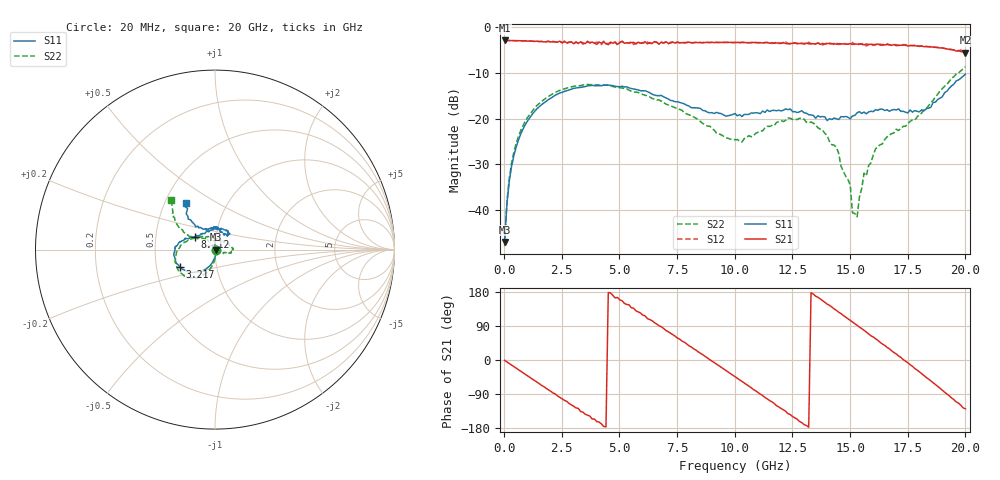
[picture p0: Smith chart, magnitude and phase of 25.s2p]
!Agilent Technologies,N5230A,US43500223,A.07.50.48
!Agilent N5230A: A.07.50.48
!Date: Sunday, September 13, 2015 17:37:15
!Correction: S11(Full 2 Port(1,2))
!S21(Full 2 Port(1,2))
!S12(Full 2 Port(1,2))
!S22(Full 2 Port(1,2))
!S2P File: Measurements: S11, S21, S12, S22:
# Hz S  dB  R 50
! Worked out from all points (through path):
!   201 points, 20 MHz to 20 GHz, reference 50 ohm
!   highest |S21| = -2.98 dB at 20 MHz (marker M1); lowest = -5.6 dB at 20 GHz (marker M2)
!   group delay of S21, straight-line fit = 116 ps
!   lowest |S11| = -46.9 dB at 20 MHz (marker M3), VSWR 1.01, Z = 50.4 - j0.124 ohm
!   |S11| at or under -10 dB: start of sweep to end of sweep
!   |S22| runs from -47.8 to -8.7 dB; largest |S21 - S12| = 0.042
!   S11 on the Smith chart (normalised r, x): 20 MHz: 1.01, -0.00; 3.217 GHz: 0.66, -0.14; 8.112 GHz: 0.79, +0.12; 20 GHz: 0.64, +0.37
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2e7  -46.90 -15.9  -2.98 -0.9  -2.97 -0.9  -47.81 -29.2
1.199e8  -38.58 -70.6  -2.98 -5.0  -2.98 -5.1  -38.16 -67.5
3.197e8  -30.45 -84.5  -3.01 -13.4  -3.00 -13.4  -29.74 -84.3
8.192e8  -22.27 -102.4  -3.07 -33.9  -3.07 -34.0  -21.53 -98.7
2.1179e9  -15.23 -133.2  -3.28 -86.9  -3.13 -86.2  -14.55 -123.2
3.2168e9  -13.25 -153.1  -3.57 -127.8  -3.68 -128.4  -12.86 -142.9
3.4166e9  -13.11 -156.6  -3.48 -137.4  -3.79 -137.6  -12.69 -145.8
5.1149e9  -12.95 177.9  -3.11 156.2  -3.21 156.1  -13.30 -175.9
6.7133e9  -15.00 159.4  -3.79 90.4  -3.71 90.0  -15.93 159.6
8.1119e9  -17.62 147.0  -3.46 34.3  -3.51 33.8  -19.35 139.9
9.011e9  -18.71 133.6  -3.37 -3.0  -3.39 -2.2  -22.13 115.1
1.001e10  -18.89 113.8  -3.41 -44.2  -3.38 -43.9  -24.59 72.1
1.15085e10  -18.46 74.0  -3.58 -107.0  -3.33 -106.4  -21.72 22.3
1.22078e10  -17.88 59.4  -3.64 -135.3  -3.28 -137.1  -20.37 6.0
1.34066e10  -19.31 48.7  -3.68 173.8  -3.89 172.7  -20.99 -13.1
1.44056e10  -20.03 63.4  -3.80 131.0  -3.52 130.8  -26.28 -20.4
1.53047e10  -18.74 74.5  -3.76 91.6  -3.97 90.4  -41.40 94.4
1.56044e10  -18.58 81.8  -3.92 78.4  -3.62 77.5  -31.91 109.4
1.67033e10  -18.40 87.8  -3.89 29.5  -3.96 28.2  -23.57 128.5
1.74026e10  -18.61 97.0  -3.97 -3.2  -3.89 -3.5  -21.67 133.4
1.85015e10  -17.53 120.2  -4.40 -55.2  -4.30 -55.5  -16.62 150.0
2e10  -10.33 121.7  -5.63 -128.8  -5.79 -129.6  -8.71 131.6
